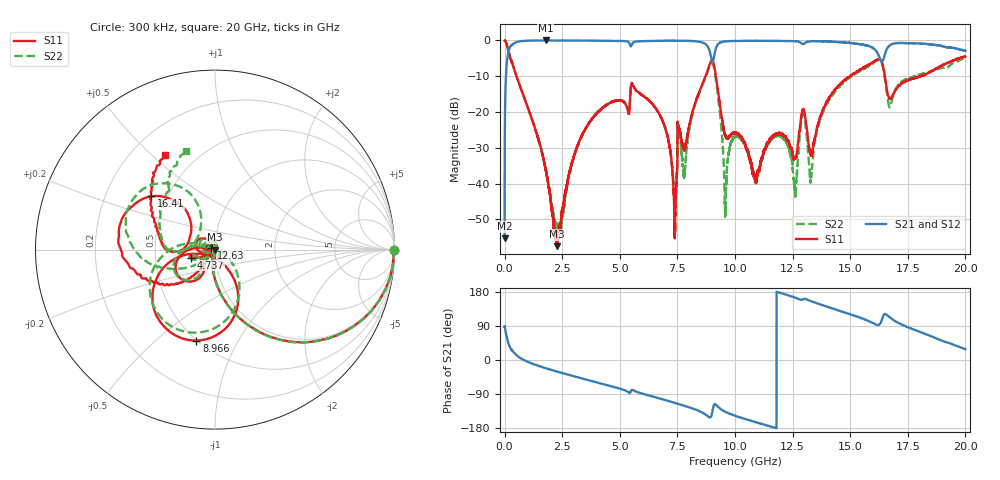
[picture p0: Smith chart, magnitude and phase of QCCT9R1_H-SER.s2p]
!{QCCT9R1}
!Johanson Technology Inc.
!www.johansontechnology.com
!Test Board Conditions:
!Substrate Type  RO4350B
!Substrate Thickness  20 mil
!Substrate Dk  3.66
!TL Type: GCPW
!TL Trace Width  34 mil
!TL Gap  10 mil
!Electrode orientation  Horizontal
!DUT TOPOLOGY	SERIES
!Mounting Pad LxW  26x52 mil
! Created Sat Jan  9 19:08:00 2021
# hz S ma R 50
! 2 Port Network Data from SP1.SP block
! freq  magS11  angS11  magS21  angS21  magS12  angS12  magS22  angS22
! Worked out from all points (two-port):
!   20001 points, 300 kHz to 20 GHz, reference 50 ohm
!   highest |S21| = 0.00 dB at 1.777 GHz (marker M1); lowest = -55.3 dB at 300 kHz (marker M2)
!   |S21| within 3 dB of the highest: 174.5 MHz to 8.901 GHz (8.727 GHz wide, 192 % of centre); 9.138 GHz to 16.14 GHz (6.998 GHz wide, 55.4 % of centre)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
!   lowest |S11| = -57.5 dB at 2.285 GHz (marker M3), VSWR 1.00, Z = 49.9 - j0.0653 ohm
!   |S11| at or under -10 dB: 515.3 MHz to 8.722 GHz (8.207 GHz wide, 178 % of centre); 9.174 GHz to 14.99 GHz (5.813 GHz wide, 48.1 % of centre); 16.51 GHz to 18.06 GHz (1.557 GHz wide, 9.01 % of centre)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
!   |S22| runs from -55.4 to 0.0 dB; largest |S21 - S12| = 0.017
!   S11 on the Smith chart (normalised r, x): 300 kHz: open; 4.737 GHz: 0.76, -0.07; 8.966 GHz: 0.50, -0.69; 12.63 GHz: 0.96, +0.02; 16.41 GHz: 0.41, +0.31; 20 GHz: 0.34, +0.55
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300000  0.9949 -0.2  0.001723 87.6  0.001778 88.9  0.9968 -0.3
1.043e8  0.8558 -32.2  0.5132 57.7  0.5142 57.5  0.8569 -32.2
2.153e8  0.622 -53.9  0.7793 35.9  0.7805 35.8  0.6228 -54.0
1.7773e9  0.01595 -108.6  0.9995 -21.5  0.9979 -21.5  0.01604 -120.7
2.2853e9  0.001339 -150.7  0.998 -30.6  0.9981 -30.6  0.002179 173.7
3.3343e9  0.04547 -146.8  0.9962 -48.3  0.9965 -48.2  0.04494 -132.2
4.7373e9  0.1413 -161.6  0.9848 -71.1  0.9854 -71.1  0.1424 -159.5
6.6673e9  0.1004 174.2  0.9887 -100.5  0.9885 -100.4  0.1001 167.9
7.3933e9  0.001931 -78.5  0.9926 -113.1  0.9923 -113.1  0.005912 -97.7
7.5993e9  0.0552 -179.9  0.9901 -116.8  0.9898 -116.8  0.04603 138.3
7.8053e9  0.02914 -118.4  0.9885 -120.8  0.9888 -120.8  0.01291 32.8
8.9663e9  0.5178 -101.6  0.5736 -148.7  0.5753 -148.8  0.4856 -108.9
9.5743e9  0.04656 -130.9  0.9706 -136.6  0.9721 -136.7  0.004128 -121.7
1.00003e10  0.05121 -75.2  0.9834 -147.0  0.9849 -147.0  0.04507 -59.1
1.08623e10  0.01178 3.5  0.9875 -163.5  0.9872 -163.5  0.01205 -153.8
1.26273e10  0.02274 156.1  0.9759 164.3  0.9752 164.3  0.007289 151.1
1.29503e10  0.1086 163.1  0.8882 160.0  0.8896 159.9  0.09351 155.9
1.33343e10  0.02494 -167.1  0.9751 154.5  0.9758 154.5  0.01629 -152.5
1.41733e10  0.1738 -129.2  0.9607 137.1  0.9648 136.9  0.1624 -144.5
1.64063e10  0.4633 140.1  0.51 112.1  0.5059 112.6  0.4428 124.4
1.66673e10  0.1621 146.1  0.8243 115.1  0.8173 115.4  0.1278 132.2
2e10  0.5968 117.8  0.7141 28.6  0.7033 28.6  0.5739 105.9
